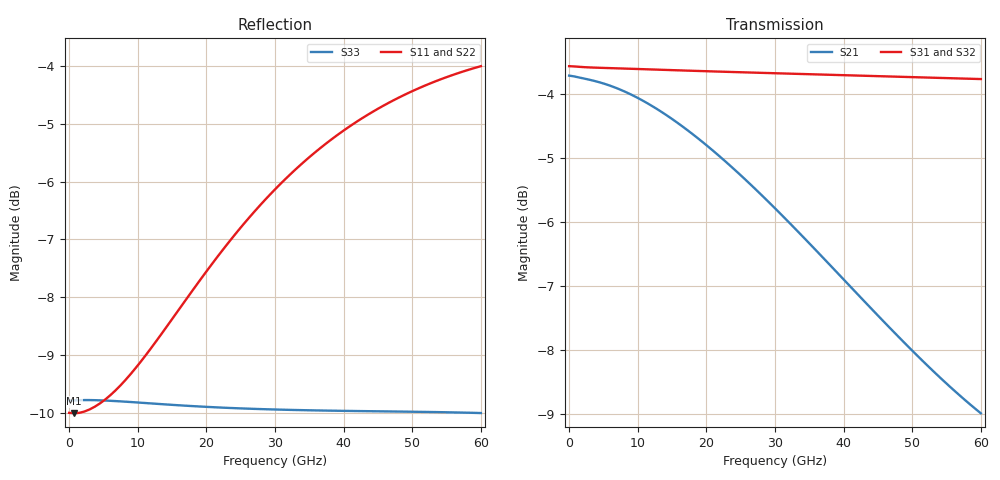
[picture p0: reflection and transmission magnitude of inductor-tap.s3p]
#  GHZ S DB R 50
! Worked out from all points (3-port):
!   82 points, 10 MHz to 60 GHz, reference 50 ohm
!   strongest paths, dB at 10 MHz, 14.25 GHz, 30 GHz, 45 GHz, 60 GHz:
!     S31: -3.6, -3.6, -3.7, -3.7, -3.8
!     S32: -3.6, -3.7, -3.7, -3.8, -3.8
!     S21: -3.7, -4.3, -5.8, -7.5, -9.0
!   lowest |S11| = -10.0 dB at 750 MHz (marker M1), VSWR 1.92, Z = 26 + j1.21 ohm
!   |S11| at or under -10 dB: 704 MHz to 795.7 MHz (91.77 MHz wide, 12.2 % of centre)
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0.01  -9.99 179.9  -3.71 -0.0  -3.56 -0.0
      -3.71 -0.0  -10.08 179.9  -3.60 -0.0
      -3.56 -0.0  -3.60 -0.0  -9.78 180.0
0.75  -10.00 176.2  -3.72 -1.9  -3.56 -0.3
      -3.72 -1.9  -10.09 176.1  -3.61 -0.3
      -3.56 -0.3  -3.61 -0.3  -9.78 179.4
7.5  -9.52 144.1  -3.93 -17.9  -3.59 -2.8
     -3.93 -17.9  -9.59 143.8  -3.64 -2.8
     -3.59 -2.8  -3.64 -2.8  -9.79 174.1
15.75  -8.25 112.0  -4.44 -36.6  -3.62 -5.7
       -4.44 -36.6  -8.29 111.4  -3.66 -5.8
       -3.62 -5.7  -3.66 -5.8  -9.86 168.0
23.25  -7.05 89.6  -5.09 -52.9  -3.65 -8.3
       -5.09 -52.9  -7.07 88.9  -3.69 -8.5
       -3.65 -8.3  -3.69 -8.5  -9.91 162.8
30.75  -6.05 71.7  -5.86 -68.8  -3.67 -11.0
       -5.86 -68.8  -6.05 70.9  -3.71 -11.1
       -3.67 -11.0  -3.71 -11.1  -9.94 157.6
37.5  -5.34 58.3  -6.61 -82.9  -3.69 -13.4
      -6.61 -82.9  -5.33 57.4  -3.73 -13.6
      -3.69 -13.4  -3.73 -13.6  -9.95 153.1
45.75  -4.69 44.2  -7.55 -100.0  -3.72 -16.3
       -7.55 -100.0  -4.68 43.2  -3.76 -16.6
       -3.72 -16.3  -3.76 -16.6  -9.97 147.6
52.5  -4.31 34.0  -8.28 -114.2  -3.74 -18.8
      -8.28 -114.2  -4.30 33.0  -3.78 -19.1
      -3.74 -18.8  -3.78 -19.1  -9.98 143.2
60  -4.01 23.8  -8.99 -130.1  -3.76 -21.7
    -8.99 -130.1  -4.00 22.6  -3.80 -22.1
    -3.76 -21.7  -3.80 -22.1  -10.00 138.4
